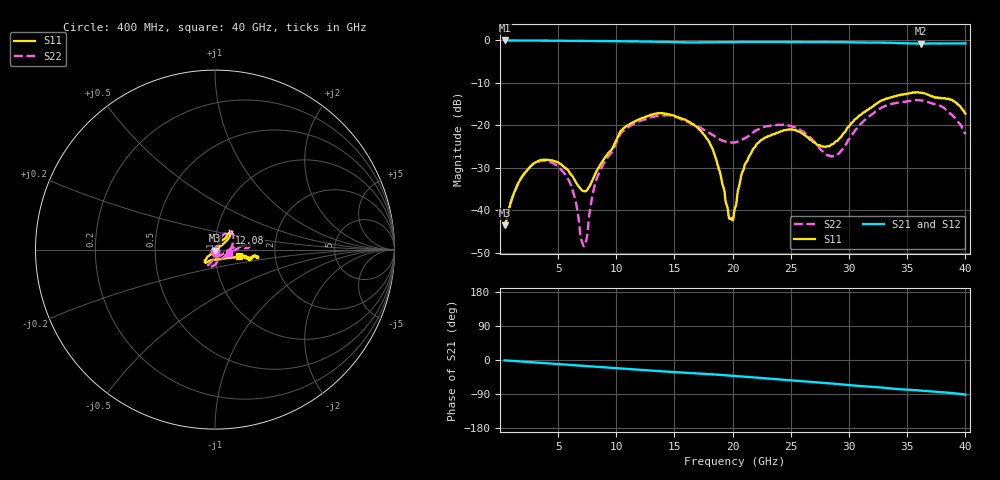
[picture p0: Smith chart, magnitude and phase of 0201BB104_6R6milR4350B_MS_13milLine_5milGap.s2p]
!Keysight Technologies,N5227A,US56070614,A.10.47.06
!Date: Wednesday, May 22, 2019 09:40:19
!Correction: S11(Full 2 Port(1,2))
!S21(Full 2 Port(1,2))
!S12(Full 2 Port(1,2))
!S22(Full 2 Port(1,2))
!S2P File: Measurements: S11, S21, S12, S22:
# Hz S  dB  R 50
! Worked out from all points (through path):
!   801 points, 400 MHz to 40 GHz, reference 50 ohm
!   highest |S21| = -0.01 dB at 400 MHz (marker M1); lowest = -0.7 dB at 36.19 GHz (marker M2)
!   group delay of S21, straight-line fit = 6.23 ps
!   lowest |S11| = -43.6 dB at 400 MHz (marker M3), VSWR 1.01, Z = 50.1 - j0.647 ohm
!   |S11| at or under -10 dB: start of sweep to end of sweep
!   |S22| runs from -48.5 to -14.1 dB; largest |S21 - S12| = 0.014
!   S11 on the Smith chart (normalised r, x): 400 MHz: 1.00, -0.01; 12.08 GHz: 1.15, +0.21; 40 GHz: 1.30, -0.09
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4e8  -43.59 -77.1  -0.01 -1.1  -0.04 -1.0  -44.03 -80.4
1.885e9  -32.18 -85.4  -0.03 -4.1  -0.03 -4.1  -32.12 -89.2
4.0135e9  -28.13 -84.9  -0.06 -8.6  -0.06 -8.6  -28.43 -97.5
5.9935e9  -31.21 -68.7  -0.08 -12.9  -0.08 -12.8  -33.41 -104.6
7.033e9  -35.30 -30.0  -0.10 -15.1  -0.10 -15.0  -47.33 -50.6
7.3795e9  -35.50 -7.4  -0.10 -15.8  -0.10 -15.8  -47.48 22.2
8.023e9  -32.49 27.9  -0.11 -17.3  -0.11 -17.2  -35.51 60.7
8.716e9  -28.92 45.2  -0.12 -18.8  -0.12 -18.7  -30.08 58.3
1.2082e10  -18.47 49.5  -0.26 -26.0  -0.26 -26.1  -18.93 55.1
1.36165e10  -17.15 46.9  -0.34 -29.3  -0.36 -29.3  -17.75 45.4
1.7527e10  -22.22 36.9  -0.46 -36.3  -0.46 -36.0  -21.11 5.5
1.8517e10  -27.57 33.0  -0.43 -38.3  -0.43 -38.0  -22.72 -14.1
1.9804e10  -41.92 -32.9  -0.38 -41.3  -0.38 -40.9  -24.04 -53.2
2.02e10  -39.44 -87.0  -0.37 -42.2  -0.37 -41.8  -24.02 -62.6
2.09425e10  -30.41 -127.3  -0.36 -43.9  -0.36 -43.4  -23.18 -77.3
2.2279e10  -23.95 -135.5  -0.37 -47.1  -0.38 -46.6  -20.84 -96.3
2.4952e10  -21.00 -128.8  -0.39 -53.3  -0.38 -52.7  -20.10 -114.0
2.6833e10  -23.64 -112.1  -0.40 -57.8  -0.39 -57.2  -23.36 -105.5
2.88625e10  -23.80 -55.0  -0.39 -63.0  -0.37 -62.5  -27.19 -49.9
3.34165e10  -13.56 -12.1  -0.53 -74.7  -0.53 -74.1  -15.12 7.8
3.61885e10  -12.28 -9.6  -0.74 -80.8  -0.72 -80.0  -14.13 6.7
4e10  -17.25 -14.3  -0.69 -91.2  -0.69 -91.2  -22.07 -14.9
